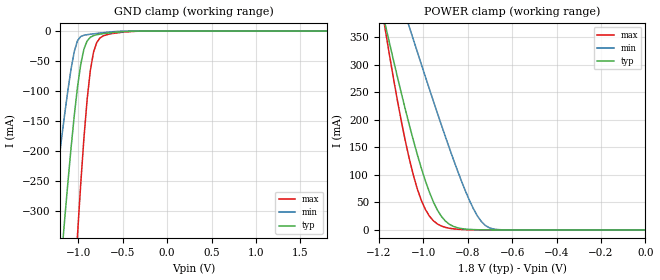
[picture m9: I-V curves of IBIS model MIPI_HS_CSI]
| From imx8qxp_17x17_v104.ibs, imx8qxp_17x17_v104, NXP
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[Model]   MIPI_HS_CSI
Model_type   Input
Polarity   Non-Inverting
Enable   Active-High
Vinh =   0.3
Vinl =   0.1
|   typ   min   max
C_comp   1.2p   1.02p   1.24p
[Temperature Range]   85   125   -40
[Voltage Range]   1.8   1.52   1.98
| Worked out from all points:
|   GND clamp passes 1 mA (typ) near -0.49 V on its own axis
|   POWER clamp passes 1 mA (typ) near -0.79 V on its own axis
[GND_clamp]
|Voltage   I (typ)   I (min)   I (max)
-1.764V   -1.504A    -927.3mA   -2.592A
-1.332V   -645.6mA   -358.9mA   -1.255A
-1.296V   -577mA     -313.1mA   -1.147A
-1.188V   -377.1mA   -180mA     -829mA
-1.152V   -313.4mA   -138.1mA   -725.8mA
-1.008V   -93.18mA   -15.98mA   -339.9mA
-972mV    -55.59mA   -9.064mA   -255.1mA
-900mV    -16.47mA   -5.99mA    -114.5mA
-864mV    -10.34mA   -5.25mA    -66mA
-792mV    -6.135mA   -3.907mA   -19.07mA
-720mV    -4.323mA   -2.673mA   -8.16mA
1.8V      4.16nA     777.7pA    57.34nA
[Power_clamp]
|Voltage   I (typ)   I (min)   I (max)
-1.782V   1.556A     1.311A     2.153A
-1.17V    371.3mA    505.9mA    361.7mA
-1.098V   247.4mA    413.6mA    196.3mA
-1.062V   189.5mA    367.9mA    127.8mA
-1.044V   162.1mA    345.2mA    98.75mA
-990mV    88.79mA    277.7mA    37mA
-918mV    24.5mA     190.3mA    7.093mA
-864mV    6.439mA    127.8mA    2.033mA
-792mV    1.021mA    53.67mA    402uA
-738mV    282.5uA    15.1mA     132.7uA
-702mV    142.9uA    3.865mA    73.38uA
0V        4.16nA     777.7pA    57.34nA
